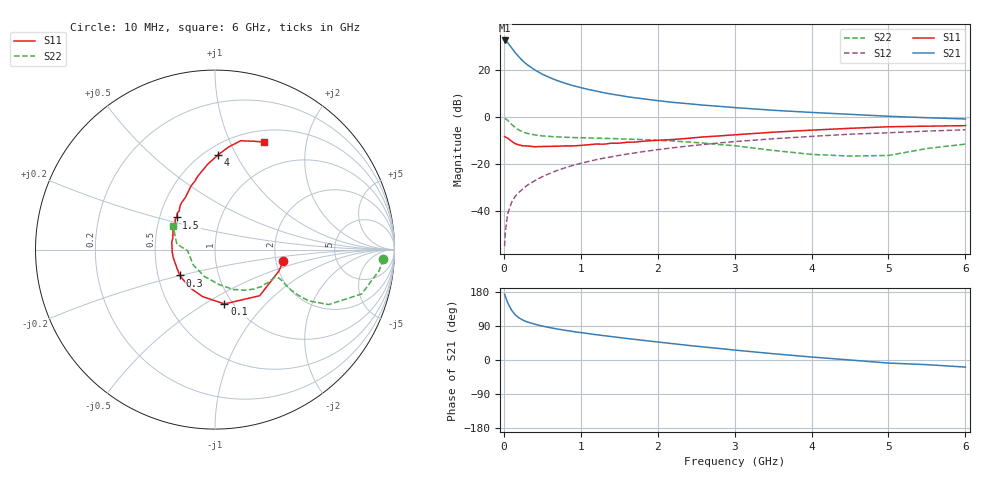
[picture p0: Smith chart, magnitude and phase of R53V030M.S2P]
! SIEMENS Small Signal Semiconductors
! BFR183
! Si NPN RF Bipolar Junction Transistor in SOT23
! VCE = 3 V  IC = 30 mA
! Common Emitter S-Parameters:  May  1996
# GHz  S  MA  R  50
!  f  S11  S21  S12  S22
! GHz  MAG  ANG  MAG  ANG  MAG  ANG  MAG  ANG
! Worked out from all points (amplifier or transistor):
!   36 points, 10 MHz to 6 GHz, reference 50 ohm
!   highest |S21| = 32.6 dB at 10 MHz (marker M1)
!   |S21| within 3 dB of that: start of sweep to 98.09 MHz
!   unconditionally stable (mu >= 1): 407.6 MHz to 2.366 GHz
!   at 250 MHz: K = 0.90, MSG = 27.1 dB, |S12| = -30.4 dB
!   at 1.4 GHz: K = 1.05, MAG = 12.0 dB, |S12| = -16.9 dB
!   at 6 GHz: K = 0.90, MSG = 2.3 dB, |S12| = -5.4 dB
!   S11 on the Smith chart (normalised r, x): 10 MHz: 2.19, -0.34; 100 MHz: 0.91, -0.61; 300 MHz: 0.65, -0.20; 1.5 GHz: 0.61, +0.24; 4 GHz: 0.58, +0.85; 6 GHz: 0.64, +1.35
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0.01  0.3865 -9.8  42.62 173.6  0.0018 94.6  0.9398 -3.3
0.02  0.3751 -18.7  42.02 167.4  0.0037 83.6  0.9219 -7.3
0.05  0.3577 -45.9  38.32 151.2  0.0088 76.0  0.8539 -16.8
0.1  0.3073 -80.2  29.89 131.6  0.0153 71.9  0.7034 -25.8
0.15  0.2707 -104.8  23.2 118.7  0.0209 70.3  0.5947 -28.7
0.2  0.2548 -121.2  18.72 110.8  0.0253 70.9  0.5262 -28.7
0.25  0.2448 -134.1  15.44 105.0  0.0301 71.5  0.4817 -28.0
0.3  0.2437 -143.7  13.16 100.7  0.0351 72.8  0.4529 -27.1
0.4  0.2343 -158.6  10.13 94.7  0.0442 73.6  0.4179 -25.3
0.5  0.2369 -169.0  8.173 89.5  0.054 74.3  0.398 -24.3
0.6  0.2386 -176.7  6.881 85.4  0.0638 73.7  0.3871 -24.0
0.7  0.24 176.1  5.938 81.6  0.0741 73.7  0.3795 -24.2
0.8  0.2442 170.4  5.214 78.3  0.084 73.0  0.3727 -24.6
0.9  0.2439 164.5  4.662 75.1  0.0943 72.3  0.3671 -25.0
1.1  0.258 155.2  3.872 69.7  0.1139 71.0  0.3605 -27.4
1.5  0.2784 139.9  2.901 59.3  0.1534 66.9  0.346 -32.6
2.2  0.3337 119.7  2.056 43.0  0.2229 59.0  0.3102 -45.1
3.5  0.4775 94.9  1.397 16.6  0.3457 42.1  0.1958 -83.5
4  0.5282 88.1  1.257 7.9  0.3891 36.0  0.1609 -111.3
4.5  0.5774 82.4  1.145 0.0  0.4324 29.1  0.1483 -144.8
5.5  0.6409 70.4  0.969 -12.3  0.5037 17.2  0.2148 171.9
6  0.6585 65.5  0.912 -18.7  0.5368 9.6  0.2661 151.0
